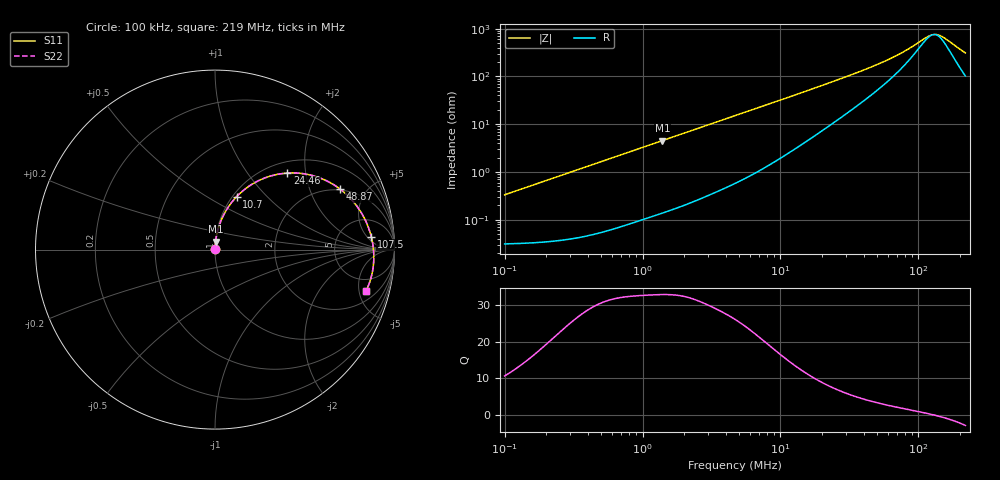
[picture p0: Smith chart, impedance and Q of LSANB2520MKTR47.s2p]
! LSANB2520MKTR47  S-PARAMETER MODEL  ( General Type )
! Model Generated by TAIYO YUDEN Corporation (http://www.ty-top.com)
! Version 2.0
! TAIYO YUDEN Control No. 20210629
! Copyright(c) 2012 TAIYO YUDEN CO.,LTD. All Rights Reserved.
! Product Description (link to TY-COMPAS)
! https://ds.yuden.co.jp/TYCOMPAS/or/detail?pn=LSANB2520MKTR47M&u=M
! Products Name : Inductors
! Characteristics :
!  Inductance : 0.47 uH , SRF(min) : -Hz , DC Resistance(max) : 0.039 Ohm
!  Rated Current : Saturation :4200 mA , Temp Rise : 3400 mA (40 degC)
!  Case Size : 2.5 x 2.0 / 0.098 x 0.079 [mm/inch] , Thickness : 1.2 / 0.047 [mm/inch]
!  (Conditions: Temperature = 25 degC , DC Bias Current/Voltage = 0A / 0V)
! External Node Assignments :
!  1  o---GGG---o  2
! GND o---------o GND
! Frequency Range : 0.1MHz  -  218.972167MHz  [ 402 STEP ]
# MHz S RI R 50
! Freq[MHz].  S11 Real  S11 Imag  S21 Real  S21 Imag  S12 Real  S12 Imag  S22 Real  S22 Imag
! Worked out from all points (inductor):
!   401 points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, 100 kHz to 219 MHz, reference 50 ohm
!   read as one part in series: L = 526 nH near 103.9 kHz
!   highest Q = 32.9 at 1.393 MHz (marker M1), where L = 517 nH
!   self-resonance near 129 MHz
!   S11 on the Smith chart (normalised r, x): 100 kHz: 1.00, +0.01; 10.7 MHz: 1.04, +0.68; 24.46 MHz: 1.22, +1.58; 48.87 MHz: 1.96, +3.30; 107.5 MHz: 11, +7; 219 MHz: 3.04, -5.88
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0.1  0.000322 0.0033  0.9997 -0.0033  0.9997 -0.0033  0.000322 0.0033
0.362673  0.000576 0.0119  0.9994 -0.0119  0.9994 -0.0119  0.000576 0.0119
1.315317  0.00311 0.0425  0.9969 -0.0425  0.9969 -0.0425  0.00311 0.0425
1.393424  0.00341 0.045  0.9966 -0.045  0.9966 -0.045  0.00341 0.045
2.731286  0.0105 0.0867  0.9895 -0.0867  0.9895 -0.0867  0.0105 0.0867
4.770297  0.0282 0.1475  0.9718 -0.1475  0.9718 -0.1475  0.0282 0.1475
7.423655  0.063 0.2198  0.937 -0.2198  0.937 -0.2198  0.063 0.2198
10.6976  0.1201 0.2946  0.8799 -0.2946  0.8799 -0.2946  0.1201 0.2946
13.47404  0.1761 0.3439  0.8239 -0.3439  0.8239 -0.3439  0.1761 0.3439
16.97108  0.2507 0.3878  0.7493 -0.3878  0.7493 -0.3878  0.2507 0.3878
24.45559  0.4023 0.4264  0.5977 -0.4264  0.5977 -0.4264  0.4023 0.4264
33.91131  0.552 0.4101  0.448 -0.4101  0.448 -0.4101  0.552 0.4101
48.86671  0.6992 0.3355  0.3008 -0.3355  0.3008 -0.3355  0.6992 0.3355
61.54953  0.7704 0.2677  0.2296 -0.2677  0.2296 -0.2677  0.7704 0.2677
80.56351  0.8307 0.1775  0.1693 -0.1775  0.1693 -0.1775  0.8307 0.1775
107.4986  0.8707 0.0718  0.1293 -0.0718  0.1293 -0.0718  0.8707 0.0718
125.3749  0.8818 0.0114  0.1182 -0.0114  0.1182 -0.0114  0.8818 0.0114
132.82  0.884 -0.012  0.116 0.012  0.116 0.012  0.884 -0.012
140.7073  0.8849 -0.036  0.1151 0.036  0.1151 0.036  0.8849 -0.036
154.9071  0.8835 -0.0769  0.1165 0.0769  0.1165 0.0769  0.8835 -0.0769
198.8997  0.8595 -0.1878  0.1405 0.1878  0.1405 0.1878  0.8595 -0.1878
218.9722  0.8411 -0.2309  0.1589 0.2309  0.1589 0.2309  0.8411 -0.2309
